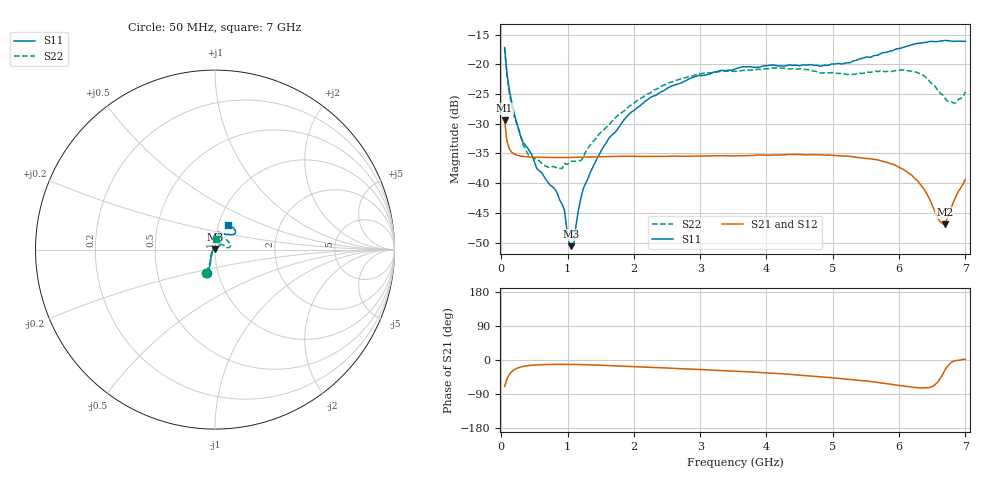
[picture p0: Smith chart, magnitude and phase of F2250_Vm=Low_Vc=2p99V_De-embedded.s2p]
! Integrated Device Technology
! Corporate Headquarters
! 6024 Silver Creek Valley Road
! San Jose, CA 95138  USA
! Phone:  1-408-284-8200
! Toll Free:  1-800-223-1366
! Webpage:  http://www.idt.com/
! Timing and RF Division
! 515 Groton Road, Suite 102
! Westford, MA 01886-6024
! Device:  F2250
! Description: Voltage Variable RF Attenuator
! Frequency:  50.0 -  6000.00 MHz
! Package:  3x3 mm Thin QFN Plastic Package: 16 pin
! Ports:  2 RF, 3 DC
!  Pin  1  = GND
!  Pin  2  = NC
!  Pin  3  = RF1  = Port 1
!  Pin  4  = NC
!  Pin  5  = GND
!  Pin  6  = GND
!  Pin  7  = GND
!  Pin  8  = GND
!  Pin  9  = NC
!  Pin 10  = RF2  = Port 2
!  Pin 11  = NC
!  Pin 12  = GND
!  Pin 13  = GND
!  Pin 14  = VCNTRL
!  Pin 15  = VDD
!  Pin 16  = VMODE
! Vcntrl:  2.990 Volts
! Vmode:  +0.000 Volts
! Vdd:  +3.30  Volts
! Current:  1.176 mA
! Data:  The device was measured on a the F2250 evaluation board which has
!  individual transmission lines to the RF pins.  Data was collected
!  using a calibrated network analyzer.  The evaluation board was
!  de-embedded using a TRL calibration technique.
!  The reference plane is the edge of the package pin.
! Misc:  SN 10
!  Action Tracker AT0258
! Date Measured:  2014-11-26
! Date:  2015-10-15  MJV
! Note:
!  Integrated Device Technology supplies this data as a sample of measured
!  data at the package pin for this product.  Your particular data for this
!  product may vary.
!  Data was taken at 25 degrees C.
!  Integrated Device Technology reserves the right to change this data at anytime.
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# GHz S dB R 50
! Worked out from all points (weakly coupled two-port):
!   201 points, 50 MHz to 7 GHz, reference 50 ohm
!   highest |S21| = -29.41 dB at 50 MHz (marker M1); lowest = -46.9 dB at 6.687 GHz (marker M2)
!   lowest |S11| = -50.6 dB at 1.058 GHz (marker M3), VSWR 1.01, Z = 49.8 + j0.247 ohm
!   |S11| at or under -10 dB: start of sweep to end of sweep
!   |S22| runs from -37.5 to -17.3 dB; largest |S21 - S12| = 6.3e-05
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0.05  -17.18 -108.6  -29.41 -69.8  -29.41 -69.8  -17.28 -111.0
0.08475  -21.45 -107.4  -32.92 -50.4  -32.92 -50.3  -21.74 -110.2
0.15425  -26.23 -116.6  -34.76 -31.1  -34.76 -31.2  -26.81 -122.5
0.29325  -32.21 -127.8  -35.44 -18.5  -35.43 -18.5  -32.11 -137.4
0.3975  -34.09 -141.8  -35.56 -15.0  -35.56 -15.0  -35.04 -160.6
0.91875  -43.53 158.0  -35.69 -11.5  -35.68 -11.5  -37.51 133.5
0.9535  -44.61 170.0  -35.68 -11.5  -35.69 -11.5  -36.64 131.2
1.023  -50.05 143.7  -35.68 -11.6  -35.67 -11.6  -36.62 116.0
1.05775  -50.59 123.0  -35.67 -11.6  -35.67 -11.6  -36.29 110.8
1.0925  -50.45 90.2  -35.66 -11.7  -35.66 -11.7  -36.30 106.4
1.162  -44.62 57.0  -35.64 -11.9  -35.64 -11.9  -36.23 95.5
1.2315  -41.08 44.3  -35.61 -12.1  -35.61 -12.1  -35.81 85.8
1.6485  -32.10 41.9  -35.52 -14.7  -35.52 -14.6  -29.87 64.6
1.96125  -28.05 42.2  -35.46 -17.2  -35.46 -17.3  -26.80 56.8
2.37825  -24.86 47.3  -35.48 -20.3  -35.48 -20.3  -23.99 56.8
3.525  -20.79 72.4  -35.41 -29.5  -35.40 -29.5  -21.19 74.7
4.7065  -20.17 72.3  -35.20 -42.6  -35.20 -42.6  -21.14 72.2
5.85325  -17.81 40.5  -36.63 -63.4  -36.64 -63.5  -21.14 23.1
6.27025  -16.50 40.0  -39.50 -72.9  -39.51 -72.9  -21.37 9.7
6.68725  -16.00 48.7  -46.89 -27.7  -46.85 -27.3  -25.63 28.7
6.861  -16.14 55.1  -42.19 -1.4  -42.15 -1.4  -26.45 57.9
7  -16.14 63.2  -39.37 1.9  -39.33 1.7  -24.63 83.0
